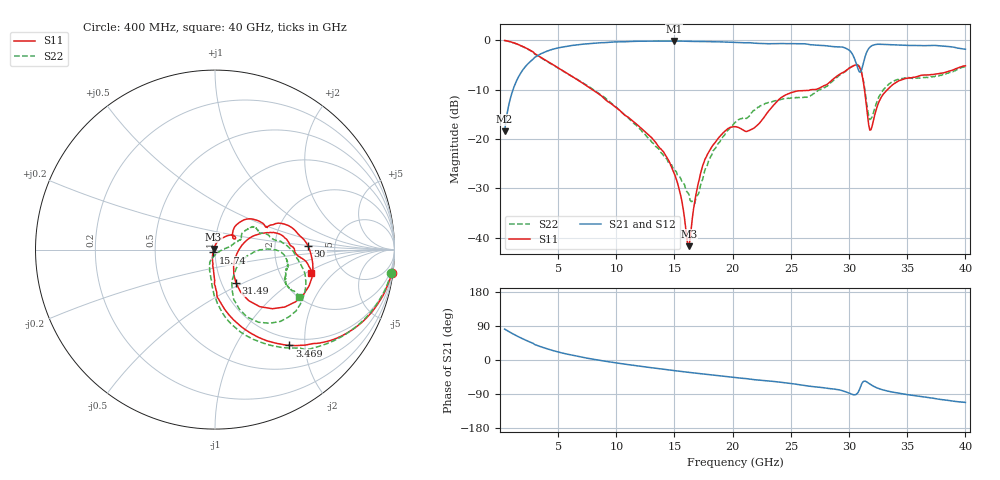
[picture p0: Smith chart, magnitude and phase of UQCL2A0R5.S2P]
! AVX Corporation
! Date:  10/27/06
! Part No:  UQCL2A0R5
! Description:  Ultra Low ESR Microwave capacitors
! Mounting Orientation:  Horizontal
# GHZ S DB R 50
! Freq  |S11|  S11 Ph  |S21|  S21 Ph  |S12|  S12 Ph  |S22|  S22 Ph
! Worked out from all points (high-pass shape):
!   401 points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, 400 MHz to 40 GHz, reference 50 ohm
!   highest |S21| = -0.18 dB at 14.95 GHz (marker M1); lowest = -18.5 dB at 400 MHz (marker M2)
!   |S21| within 3 dB of the highest: 3.2 GHz to 30.36 GHz (27.16 GHz wide, 162 % of centre); 31.4 GHz to end of sweep
!   lowest |S11| = -41.7 dB at 16.24 GHz (marker M3), VSWR 1.02, Z = 49.2 + j0.312 ohm
!   |S11| at or under -10 dB: 7.931 GHz to 26.83 GHz (18.9 GHz wide, 109 % of centre); 26.93 GHz to 27.08 GHz (148.5 MHz wide, 0.55 % of centre); 31.32 GHz to 33.31 GHz (1.985 GHz wide, 6.14 % of centre)
!   |S22| runs from -33.1 to -0.1 dB; largest |S21 - S12| = 0.0065
!   S11 on the Smith chart (normalised r, x): 400 MHz: 1, -15; 3.469 GHz: 0.87, -1.70; 15.74 GHz: 0.98, -0.03; 30 GHz: 3.15, +0.18; 31.49 GHz: 1.17, -0.46; 40 GHz: 3.00, -1.10
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0.4  -0.06 -7.7  -18.47 81.6  -18.48 81.6  -0.10 -7.5
1.489  -0.79 -26.4  -7.92 62.9  -7.93 62.9  -0.83 -26.5
3.469  -3.40 -52.1  -2.82 35.4  -2.83 35.5  -3.46 -54.5
7.033  -8.60 -77.9  -0.84 7.5  -0.84 7.6  -8.51 -81.8
13.666  -21.64 -98.1  -0.18 -22.9  -0.18 -22.9  -22.08 -112.1
14.953  -26.79 -107.8  -0.18 -27.9  -0.17 -27.9  -26.15 -108.0
15.745  -34.15 -125.6  -0.20 -30.9  -0.19 -30.9  -29.00 -95.8
16.24  -41.71 157.3  -0.24 -32.7  -0.23 -32.8  -31.20 -82.0
16.834  -31.38 83.2  -0.26 -34.8  -0.25 -34.8  -32.05 -31.5
17.626  -24.09 64.5  -0.27 -37.5  -0.26 -37.5  -26.23 2.9
20.2  -17.51 31.3  -0.45 -46.3  -0.44 -46.4  -16.66 21.2
21.586  -18.09 38.0  -0.54 -51.0  -0.53 -51.1  -14.81 31.6
24.259  -11.49 39.9  -0.68 -59.3  -0.67 -59.4  -11.96 30.2
26.833  -10.00 23.0  -0.95 -69.8  -0.94 -70.0  -11.04 19.0
28.714  -7.74 20.4  -1.32 -76.8  -1.32 -76.9  -8.02 3.6
30.001  -5.69 2.3  -2.01 -87.1  -2.01 -87.2  -5.66 -15.5
30.496  -5.07 -12.0  -3.90 -91.9  -3.91 -92.0  -5.03 -29.1
30.892  -5.43 -32.8  -6.44 -78.2  -6.45 -78.4  -5.33 -47.6
31.486  -13.12 -58.0  -2.61 -57.1  -2.63 -57.4  -12.22 -67.0
31.882  -18.14 -11.3  -1.24 -65.2  -1.26 -65.5  -15.93 -27.8
33.466  -9.64 16.7  -0.91 -83.0  -0.93 -83.2  -8.81 -2.1
40  -5.19 -13.5  -1.84 -112.0  -1.86 -112.3  -5.38 -29.3
